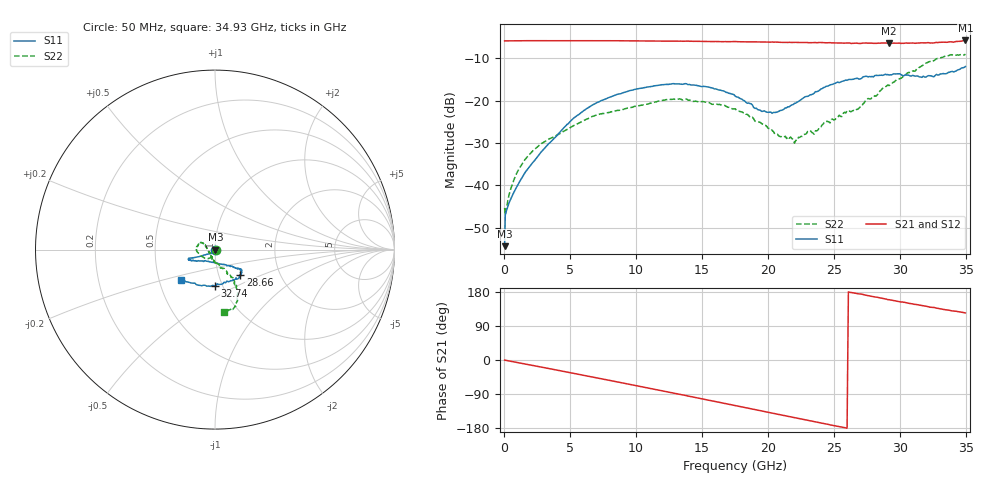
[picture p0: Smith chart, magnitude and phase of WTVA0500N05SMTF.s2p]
! 50 ohm 2-Port S-parameters measured by Modelithics Inc support@modelithics.com  Tampa, FL USA 813-866-6335 (February 2024)
! Smiths Interconnect,  5dB P/N: WTVA0500N05SMTF, Temperature: 0 C
! Board: 10 mil Rogers 4350B, Mounting Pad Dimensions: Length: 15 mils, Width: 25 mils, Gap: 40 mils.
# Hz S RI R 50
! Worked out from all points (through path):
!   352 points, 50 MHz to 34.93 GHz, reference 50 ohm
!   highest |S21| = -5.82 dB at 34.93 GHz (marker M1); lowest = -6.5 dB at 29.15 GHz (marker M2)
!   group delay of S21, straight-line fit = 19.1 ps
!   lowest |S11| = -54.4 dB at 50 MHz (marker M3), VSWR 1.00, Z = 50.2 + j0.00575 ohm
!   |S11| at or under -10 dB: start of sweep to end of sweep
!   |S22| runs from -47.0 to -9.1 dB; largest |S21 - S12| = 0.0033
!   S11 on the Smith chart (normalised r, x): 50 MHz: 1.00, +0.00; 28.66 GHz: 1.27, -0.37; 32.74 GHz: 0.92, -0.39; 34.93 GHz: 0.65, -0.23
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5e7  0.00191 5.73e-05  0.5059 -0.00255  0.5058 -0.00288  0.0054 0.000107
1e8  0.00433 -0.00107  0.5059 -0.00544  0.5057 -0.00553  0.00396 -0.0021
4.985e8  0.00277 -0.00619  0.5058 -0.028  0.5056 -0.0281  0.00343 -0.00822
1.0955e9  -0.000821 -0.0104  0.5038 -0.0629  0.5035 -0.0629  0.00125 -0.0151
2.787e9  -0.0147 -0.0195  0.4821 -0.1605  0.4817 -0.1606  -0.00252 -0.0305
5.8715e9  -0.0651 -0.032  0.3943 -0.3225  0.3939 -0.3225  -0.0302 -0.0476
8.558e9  -0.1097 -0.0434  0.2716 -0.4287  0.271 -0.4287  -0.0613 -0.0454
1.1742e10  -0.1439 -0.0486  0.0897 -0.4957  0.0889 -0.4955  -0.0977 -0.0144
1.52245e10  -0.1325 -0.0625  -0.123 -0.4826  -0.1233 -0.4822  -0.0905 0.0322
1.7513e10  -0.0942 -0.0613  -0.2505 -0.4288  -0.2508 -0.4283  -0.07 0.0383
2.0299e10  -0.0119 -0.0696  -0.3759 -0.3155  -0.3759 -0.3149  -0.0437 0.00681
2.1692e10  0.0325 -0.0806  -0.4197 -0.2436  -0.4197 -0.2431  -0.0341 -0.0143
2.19905e10  0.0419 -0.0825  -0.4301 -0.2291  -0.43 -0.2285  -0.027 -0.016
2.29855e10  0.0686 -0.0885  -0.4503 -0.172  -0.4501 -0.1717  -0.0254 -0.0349
2.33835e10  0.0784 -0.0899  -0.4588 -0.1527  -0.4587 -0.1522  -0.0228 -0.0344
2.4279e10  0.1046 -0.098  -0.4699 -0.0979  -0.4697 -0.0975  -0.0167 -0.0539
2.5274e10  0.125 -0.1075  -0.4772 -0.0412  -0.4769 -0.041  -0.005 -0.0639
2.67665e10  0.142 -0.1151  -0.4721 0.0425  -0.4717 0.0429  0.0141 -0.0775
2.8657e10  0.1405 -0.1396  -0.4548 0.1428  -0.4545 0.1429  0.0659 -0.1229
2.91545e10  0.1353 -0.1468  -0.4405 0.168  -0.4399 0.1686  0.0668 -0.1344
3.27365e10  -0.00131 -0.2034  -0.355 0.3312  -0.3551 0.3305  0.126 -0.2847
3.49255e10  -0.1889 -0.1667  -0.2879 0.423  -0.2857 0.424  0.0486 -0.3481
